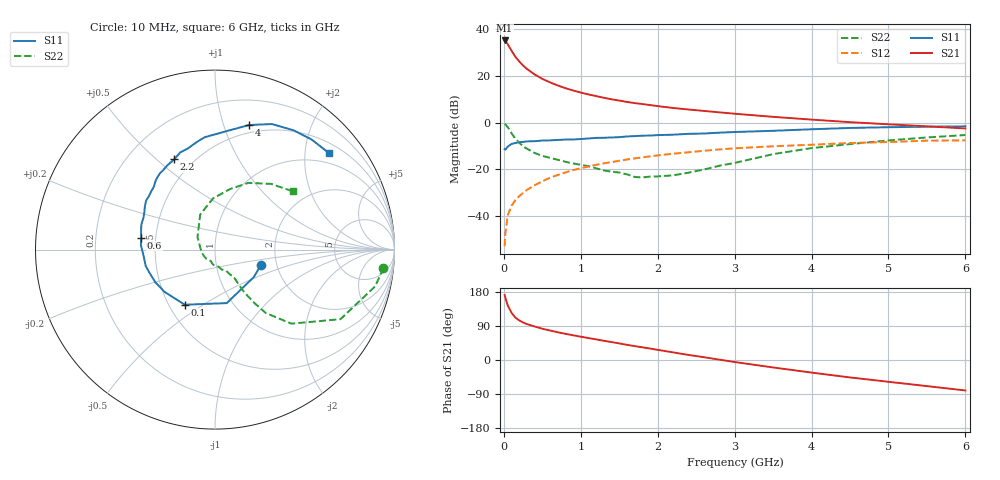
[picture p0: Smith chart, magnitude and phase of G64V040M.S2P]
! SIEMENS Small Signal Semiconductors
! BFG193
! Si NPN RF Bipolar Junction Transistor in SOT223
! VCE = 4 V  IC = 40 mA
! Common Emitter S-Parameters:  August  1996
# GHz  S  MA  R  50
!  f  S11  S21  S12  S22
! GHz  MAG  ANG  MAG  ANG  MAG  ANG  MAG  ANG
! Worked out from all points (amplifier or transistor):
!   36 points, 10 MHz to 6 GHz, reference 50 ohm
!   highest |S21| = 35.1 dB at 10 MHz (marker M1)
!   |S21| within 3 dB of that: start of sweep to 75.45 MHz
!   unconditionally stable (mu >= 1): 493.2 MHz to 2.467 GHz
!   at 250 MHz: K = 0.89, MSG = 27.2 dB, |S12| = -30.0 dB
!   at 1.4 GHz: K = 1.04, MAG = 12.1 dB, |S12| = -16.9 dB
!   at 6 GHz: K = 0.89, MSG = 2.5 dB, |S12| = -7.6 dB
!   S11 on the Smith chart (normalised r, x): 10 MHz: 1.65, -0.31; 100 MHz: 0.60, -0.42; 600 MHz: 0.41, +0.07; 2.2 GHz: 0.40, +0.57; 4 GHz: 0.42, +1.22; 6 GHz: 0.72, +2.54
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0.01  0.2695 -18.6  56.61 171.5  0.0023 88.7  0.9431 -6.2
0.02  0.265 -35.4  54.73 164.4  0.0043 83.1  0.9166 -12.8
0.05  0.3052 -77.6  47.14 144.3  0.0105 71.4  0.7995 -29.0
0.1  0.3501 -118.7  34.27 124.5  0.0167 67.1  0.5931 -44.1
0.15  0.3665 -139.8  25.41 111.8  0.022 64.3  0.4527 -51.3
0.2  0.379 -151.2  20.15 104.5  0.0269 65.7  0.3724 -53.5
0.25  0.3871 -160.5  16.5 99.0  0.0315 66.6  0.3117 -54.9
0.3  0.3967 -166.6  13.96 94.7  0.0366 67.3  0.2769 -55.7
0.4  0.4001 -175.8  10.67 88.5  0.0461 67.9  0.2247 -55.7
0.5  0.4137 176.6  8.576 82.5  0.0558 67.1  0.1948 -55.5
0.6  0.4168 170.7  7.209 77.8  0.0664 66.4  0.1766 -56.7
0.8  0.4336 161.1  5.427 69.1  0.0861 63.4  0.1457 -60.7
1.1  0.4582 148.5  3.988 57.9  0.1154 58.5  0.1168 -71.4
1.3  0.4734 141.0  3.387 50.7  0.1349 54.6  0.0953 -79.9
1.6  0.5055 131.0  2.756 40.0  0.1629 47.9  0.0787 -101.9
2.2  0.5515 114.3  2.049 20.1  0.2162 34.5  0.0747 -165.3
2.8  0.6085 99.5  1.653 1.0  0.2669 20.5  0.1198 144.4
3.5  0.6674 83.5  1.325 -19.7  0.3119 3.3  0.212 112.9
4  0.7196 74.7  1.158 -33.2  0.336 -6.4  0.2851 92.3
4.5  0.7681 65.6  1.021 -46.0  0.3662 -16.6  0.3469 76.2
5.5  0.8161 48.7  0.832 -68.9  0.4111 -39.9  0.4815 49.5
6  0.8319 40.4  0.749 -80.4  0.4172 -53.2  0.5424 36.7
